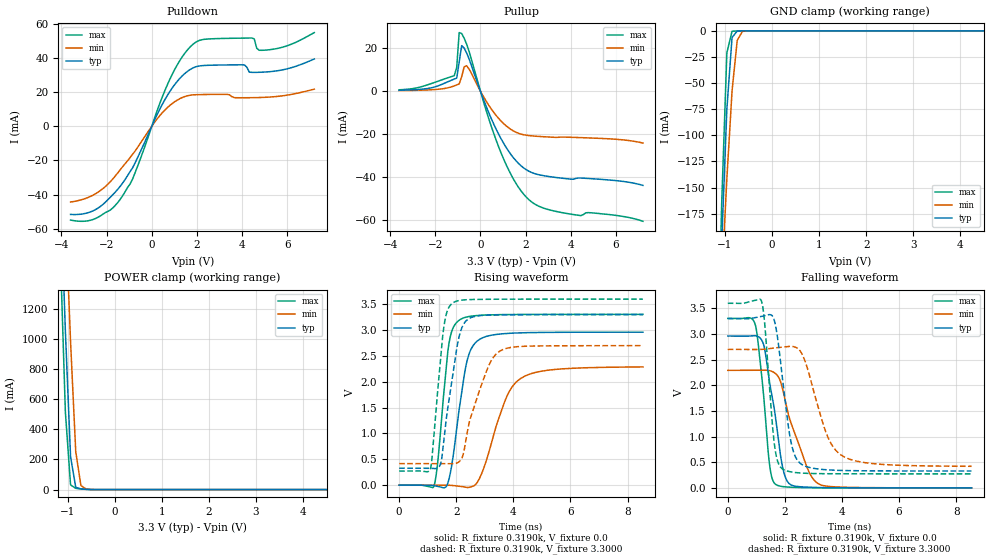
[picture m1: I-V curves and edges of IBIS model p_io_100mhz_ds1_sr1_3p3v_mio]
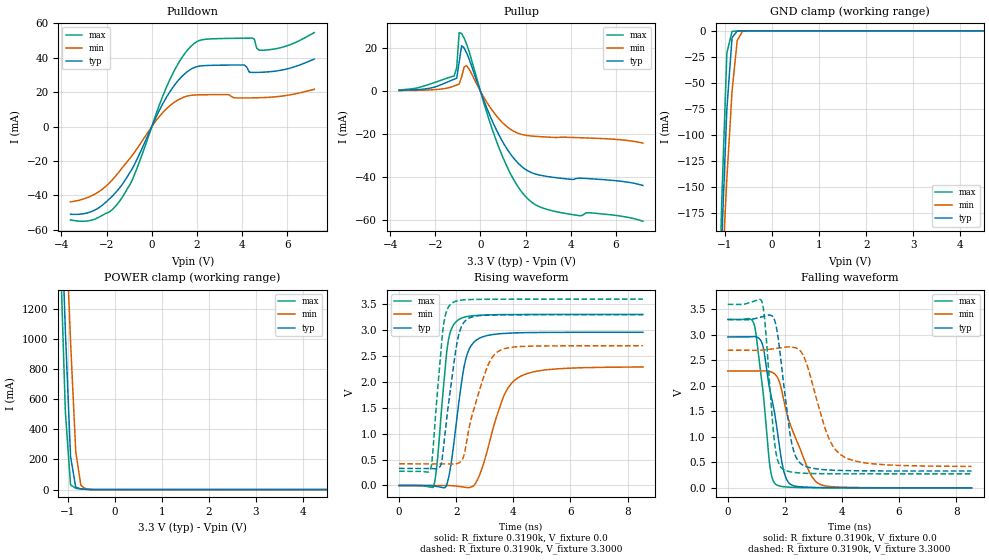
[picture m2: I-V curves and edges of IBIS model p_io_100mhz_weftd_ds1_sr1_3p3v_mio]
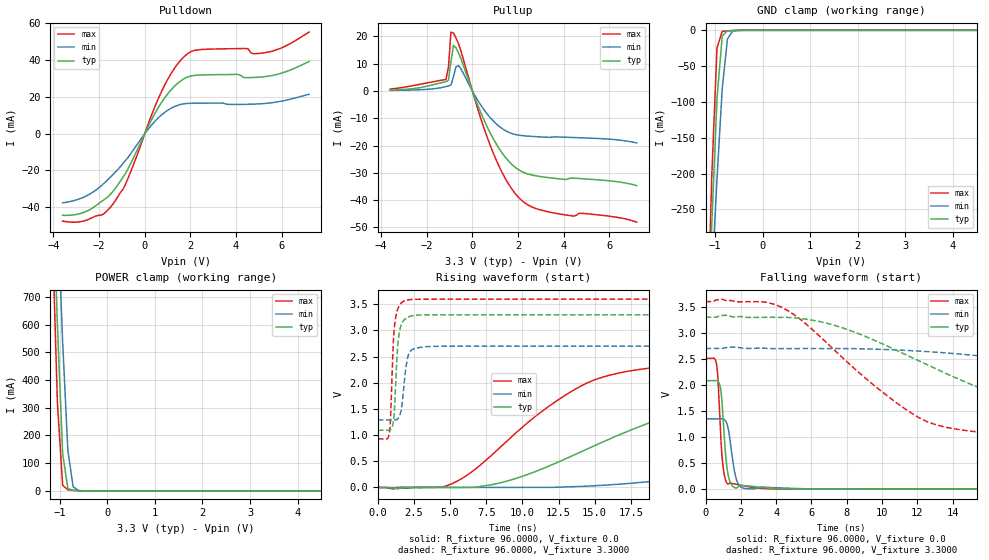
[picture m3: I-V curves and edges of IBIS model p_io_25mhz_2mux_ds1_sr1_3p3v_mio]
| IBIS file was generated by Viper version: 2025.10.06
[IBIS Ver]   6.0
[Comment Char]   |_char
[File Name]   c15x_c05x_32qfn.ibs
[File Rev]   1.0
[Date]   Wed Oct 22 17:23:39 2025
[Source]   NXP Viper 2025.10.06
[Notes]
[Disclaimer] IMPORTANT NOTICE
  This information is provided on an AS IS basis and without warranty.
  IN NO EVENT SHALL NXP BE LIABLE FOR INCIDENTAL OR CONSEQUENTIAL
  DAMAGES ARISING FROM USE OF THIS INFORMATION. THIS DISCLAIMER OF
  WARRANTY EXTENDS TO THE USER OF THE INFORMATION, AND TO THEIR CUSTOMERS
  OR USERS OF PRODUCTS  AND IS IN LIEU OF ALL WARRANTIES WHETHER EXPRESS,
  IMPLIED, OR STATUTORY, INCLUDING IMPLIED WARRANTIES OF MERCHANTABILITY
  OR FITNESS FOR PARTICULAR PURPOSE.
  NXP does not represent or warrant that the information furnished
  hereunder is free of infringement of any third party patents,
  copyrights, trade secrets, or other intellectual property rights.
  NXP does not represent or warrant that the information is free of
  defect, or that it meets any particular standard, requirements or need
  of the user of the infomation or their customers.
  NXP reserves the right to change the information in this file
  without notice.
   http://www.nxp.com
[Copyright]   (C) Copyright NXP 2004 - 2025, All Rights Reserved.
|   C15x_C05x_32QFN
[Component]   C15x_C05x_32QFN
[Manufacturer]   NXP
[Package]
| variable   typ   min   max
R_pkg   0.17548   0.155   0.21262
L_pkg   1.829e-09   1.531e-09   2.180e-09
C_pkg   1.363e-13   1.228e-13   1.594e-13
[Pin] signal_name   model_name   R_pin   L_pin   C_pin
1   P1_8   a_ip_io_3v_3p3v   0.19586   2.033e-09 1.444e-13
2   P1_9   a_ip_io_3v_3p3v   0.16891   1.839e-09 1.304e-13
3   P1_29   a_ip_io_3v_3p3v   0.15743   1.690e-09 1.249e-13
4   P1_30   a_ip_io_3v_3p3v   0.1554   1.610e-09 1.266e-13
5   P1_31   a_ip_io_3v_3p3v   0.1671   1.531e-09 1.394e-13
6   VDD_ANA   POWER   NA   NA   NA
7   VDD   POWER   NA   NA   NA
8   P2_2   a_ip_io_3v_3p3v   0.20204   2.076e-09 1.443e-13
9   P2_3   a_ip_io_3v_3p3v   0.18652   2.023e-09 1.375e-13
10   P2_7   a_ip_io_3v_3p3v   0.17002   1.817e-09 1.358e-13
11   P2_12   a_ip_io_3v_3p3v   0.16167   1.626e-09 1.309e-13
12   P2_13   a_ip_io_3v_3p3v   0.16236   1.566e-09 1.312e-13
13   P2_16   a_ip_io_3v_3p3v   0.16285   1.730e-09 1.317e-13
14   P2_17   a_ip_io_3v_3p3v   0.17748   1.921e-09 1.354e-13
15   P3_29   a_ip_io_3v_3p3v   0.17976   1.975e-09 1.316e-13
16   P3_28   a_ip_io_3v_3p3v   0.1962   2.019e-09 1.412e-13
17   P3_27   a_ip_io_3v_3p3v   0.21262   1.982e-09 1.525e-13
18   P3_11   a_ip_io_3v_3p3v   0.20043   2.180e-09 1.461e-13
19   P3_10   a_ip_io_3v_3p3v   0.17928   1.961e-09 1.401e-13
20   P3_9   a_ip_io_3v_3p3v   0.16389   1.788e-09 1.317e-13
21   P3_8   a_ip_io_3v_3p3v   0.1552   1.677e-09 1.278e-13
22   P3_1   a_ip_io_3v_3p3v   0.15887   1.668e-09 1.301e-13
23   P3_0   a_ip_io_3v_3p3v   0.1749   1.596e-09 1.442e-13
24   VDD   POWER   NA   NA   NA
25   P0_0   a_ip_io_3v_3p3v   0.19842   2.035e-09 1.483e-13
26   P0_1   a_ip_io_3v_3p3v   0.17716   1.923e-09 1.400e-13
27   P0_2   a_ip_io_3v_3p3v   0.1611   1.762e-09 1.312e-13
28   P0_3   a_ip_io_3v_3p3v   0.15523   1.732e-09 1.229e-13
29   P1_0   a_ip_io_3v_3p3v   0.155   1.701e-09 1.228e-13
30   P1_1   a_ip_io_3v_3p3v   0.16149   1.745e-09 1.302e-13
31   P1_2   a_ip_io_3v_3p3v   0.17972   1.876e-09 1.400e-13
32   P1_3   a_ip_io_3v_3p3v   0.21209   1.954e-09 1.594e-13
33   VSS   GND   NA   NA   NA
[Pin Mapping]   pulldown_ref   pullup_ref
1   VSS   VDD
2   VSS   VDD
3   VSS   VDD
4   VSS   VDD
5   VSS   VDD
6   NC   VDD_ANA
7   NC   VDD
8   VSS   VDD
9   VSS   VDD
10   VSS   VDD
11   VSS   VDD
12   VSS   VDD
13   VSS   VDD
14   VSS   VDD
15   VSS   VDD
16   VSS   VDD
17   VSS   VDD
18   VSS   VDD
19   VSS   VDD
20   VSS   VDD
21   VSS   VDD
22   VSS   VDD
23   VSS   VDD
24   NC   VDD
25   VSS   VDD
26   VSS   VDD
27   VSS   VDD
28   VSS   VDD
29   VSS   VDD
30   VSS   VDD
31   VSS   VDD
32   VSS   VDD
33   VSS   NC
|*   Model Selector   *
[Model Selector] a_ip_io_3v_3p3v
p_io_25mhz_ds0_sr0_3p3v_mio   dse=0 sre=0 25mhz
p_io_25mhz_ds0_sr1_3p3v_mio   dse=0 sre=1 25mhz
p_io_25mhz_ds1_sr0_3p3v_mio   dse=1 sre=0 25mhz
p_io_25mhz_ds1_sr1_3p3v_mio   dse=1 sre=1 25mhz
p_io_25mhz_r40_ds0_sr0_3p3v_mio   dse=0 sre=0 25mhz_r40
p_io_25mhz_r40_ds0_sr1_3p3v_mio   dse=0 sre=1 25mhz_r40
p_io_25mhz_r40_ds1_sr0_3p3v_mio   dse=1 sre=0 25mhz_r40
p_io_25mhz_r40_ds1_sr1_3p3v_mio   dse=1 sre=1 25mhz_r40
p_io_50mhz_ds0_sr0_3p3v_mio   dse=0 sre=0 50mhz
p_io_50mhz_ds0_sr1_3p3v_mio   dse=0 sre=1 50mhz
p_io_50mhz_ds1_sr0_3p3v_mio   dse=1 sre=0 50mhz
p_io_50mhz_ds1_sr1_3p3v_mio   dse=1 sre=1 50mhz
p_io_25mhz_cap_ds0_sr0_3p3v_mio   dse=0 sre=0 25mhz_cap
p_io_25mhz_cap_ds0_sr1_3p3v_mio   dse=0 sre=1 25mhz_cap
p_io_25mhz_cap_ds1_sr0_3p3v_mio   dse=1 sre=0 25mhz_cap
p_io_25mhz_cap_ds1_sr1_3p3v_mio   dse=1 sre=1 25mhz_cap
p_io_25mhz_2mux_ds0_sr0_3p3v_mio   dse=0 sre=0 25mhz_2mux
p_io_25mhz_2mux_ds0_sr1_3p3v_mio   dse=0 sre=1 25mhz_2mux
p_io_25mhz_2mux_ds1_sr0_3p3v_mio   dse=1 sre=0 25mhz_2mux
p_io_25mhz_2mux_ds1_sr1_3p3v_mio   dse=1 sre=1 25mhz_2mux
p_io_100mhz_ds0_sr0_3p3v_mio   dse=0 sre=0 100mhz
p_io_100mhz_ds0_sr1_3p3v_mio   dse=0 sre=1 100mhz
p_io_100mhz_ds1_sr0_3p3v_mio   dse=1 sre=0 100mhz
p_io_100mhz_ds1_sr1_3p3v_mio   dse=1 sre=1 100mhz
p_io_100mhz_weftd_ds0_sr0_3p3v_mio   dse=0 sre=0 100mhz
p_io_100mhz_weftd_ds0_sr1_3p3v_mio   dse=0 sre=1 100mhz
p_io_100mhz_weftd_ds1_sr0_3p3v_mio   dse=1 sre=0 100mhz
p_io_100mhz_weftd_ds1_sr1_3p3v_mio   dse=1 sre=1 100mhz
p_io_i2c_ds00_ds10_sr0_3p3v_mio   dse0=0 dse1=0 sre=0 i2c
p_io_i2c_ds00_ds10_sr1_3p3v_mio   dse0=0 dse1=0 sre=1 i2c
p_io_i2c_ds00_ds11_sr0_3p3v_mio   dse0=0 dse1=1 sre=0 i2c
p_io_i2c_ds00_ds11_sr1_3p3v_mio   dse0=0 dse1=1 sre=1 i2c
p_io_i2c_ds01_ds10_sr0_3p3v_mio   dse0=1 dse1=0 sre=0 i2c
p_io_i2c_ds01_ds10_sr1_3p3v_mio   dse0=1 dse1=0 sre=1 i2c
p_io_i2c_ds01_ds11_sr0_3p3v_mio   dse0=1 dse1=1 sre=0 i2c
p_io_i2c_ds01_ds11_sr1_3p3v_mio   dse0=1 dse1=1 sre=1 i2c
p_io_i2c_i2c1_3p3v_mio   ipp_i2c_lv=1 i2c
p_io_i2cfmp_ds00_ds10_sr0_3p3v_mio   dse0=0 dse1=0 sre=0 i2cfmp
p_io_i2cfmp_ds00_ds10_sr1_3p3v_mio   dse0=0 dse1=0 sre=1 i2cfmp
p_io_i2cfmp_ds00_ds11_sr0_3p3v_mio   dse0=0 dse1=1 sre=0 i2cfmp
p_io_i2cfmp_ds00_ds11_sr1_3p3v_mio   dse0=0 dse1=1 sre=1 i2cfmp
p_io_i2cfmp_ds01_ds10_sr0_3p3v_mio   dse0=1 dse1=0 sre=0 i2cfmp
p_io_i2cfmp_ds01_ds10_sr1_3p3v_mio   dse0=1 dse1=0 sre=1 i2cfmp
p_io_i2cfmp_ds01_ds11_sr0_3p3v_mio   dse0=1 dse1=1 sre=0 i2cfmp
p_io_i2cfmp_ds01_ds11_sr1_3p3v_mio   dse0=1 dse1=1 sre=1 i2cfmp
p_io_i2cfmp_i2c1_3p3v_mio   ipp_i2c_lv=1 i2cfmp
p_io_rst_3p3v_mio   rst
p_io_rst_rx1p8v_3p3v_mio   rst
p_io_aon_3p3v_mio   rst
| End [Component] C15x_C05x_32QFN
| Models and submodels in the file (49): p_io_100mhz_ds0_sr0_3p3v_mio (I/O), p_io_100mhz_ds0_sr1_3p3v_mio (I/O), p_io_100mhz_ds1_sr0_3p3v_mio (I/O), p_io_100mhz_ds1_sr1_3p3v_mio (I/O), p_io_100mhz_weftd_ds0_sr0_3p3v_mio (I/O), p_io_100mhz_weftd_ds0_sr1_3p3v_mio (I/O), p_io_100mhz_weftd_ds1_sr0_3p3v_mio (I/O), p_io_100mhz_weftd_ds1_sr1_3p3v_mio (I/O), p_io_25mhz_2mux_ds0_sr0_3p3v_mio (I/O), p_io_25mhz_2mux_ds0_sr1_3p3v_mio (I/O), p_io_25mhz_2mux_ds1_sr0_3p3v_mio (I/O), p_io_25mhz_2mux_ds1_sr1_3p3v_mio (I/O), p_io_25mhz_cap_ds0_sr0_3p3v_mio (I/O), p_io_25mhz_cap_ds0_sr1_3p3v_mio (I/O), p_io_25mhz_cap_ds1_sr0_3p3v_mio (I/O), p_io_25mhz_cap_ds1_sr1_3p3v_mio (I/O), p_io_25mhz_ds0_sr0_3p3v_mio (I/O), p_io_25mhz_ds0_sr1_3p3v_mio (I/O), p_io_25mhz_ds1_sr0_3p3v_mio (I/O), p_io_25mhz_ds1_sr1_3p3v_mio (I/O), p_io_25mhz_r40_ds0_sr0_3p3v_mio (I/O), p_io_25mhz_r40_ds0_sr1_3p3v_mio (I/O), p_io_25mhz_r40_ds1_sr0_3p3v_mio (I/O), p_io_25mhz_r40_ds1_sr1_3p3v_mio (I/O), p_io_50mhz_ds0_sr0_3p3v_mio (I/O), p_io_50mhz_ds0_sr1_3p3v_mio (I/O), p_io_50mhz_ds1_sr0_3p3v_mio (I/O), p_io_50mhz_ds1_sr1_3p3v_mio (I/O), p_io_aon_3p3v_mio (I/O), p_io_i2c_ds00_ds10_sr0_3p3v_mio (I/O), p_io_i2c_ds00_ds10_sr1_3p3v_mio (I/O), p_io_i2c_ds00_ds11_sr0_3p3v_mio (I/O), p_io_i2c_ds00_ds11_sr1_3p3v_mio (I/O), p_io_i2c_ds01_ds10_sr0_3p3v_mio (I/O), p_io_i2c_ds01_ds10_sr1_3p3v_mio (I/O), p_io_i2c_ds01_ds11_sr0_3p3v_mio (I/O), p_io_i2c_ds01_ds11_sr1_3p3v_mio (I/O), p_io_i2c_i2c1_3p3v_mio (I/O), p_io_i2cfmp_ds00_ds10_sr0_3p3v_mio (I/O), p_io_i2cfmp_ds00_ds10_sr1_3p3v_mio (I/O), p_io_i2cfmp_ds00_ds11_sr0_3p3v_mio (I/O), p_io_i2cfmp_ds00_ds11_sr1_3p3v_mio (I/O), p_io_i2cfmp_ds01_ds10_sr0_3p3v_mio (I/O), p_io_i2cfmp_ds01_ds10_sr1_3p3v_mio (I/O), p_io_i2cfmp_ds01_ds11_sr0_3p3v_mio (I/O), p_io_i2cfmp_ds01_ds11_sr1_3p3v_mio (I/O), p_io_i2cfmp_i2c1_3p3v_mio (I/O), p_io_rst_3p3v_mio (I/O), p_io_rst_rx1p8v_3p3v_mio (I/O)
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[Model] p_io_100mhz_ds1_sr1_3p3v_mio
|   Model p_io_100mhz_ds1_sr1_3p3v_mio
| This model was characterised for following simulation conditions:
| External (pad) voltage:
|   - Typ: 3.3V,   - Min: 2.7V,   - Max: 3.6V
| Library cells for typ/min/max conditions are connected as defined below:
|  pad - External Pad
|  ipp_do_lv - Core Input
|  ipp_obe_lv - Output Buffer Enable
|  IOGC - NC
|  REFH3V3 - REFH3V3
|  REFL3V3 - REFL3V3
|  ZI - NC
|  abut_ncal_vddio[1] - vddio
|  abut_ncal_vddio[2] - vddio
|  abut_ncal_vddio[3] - vssio
|  abut_ncal_vddio[4] - vddio
|  abut_ncal_vddio[5] - vddio
|  abut_ncal_vddio[6] - vssio
|  abut_pcal_vddio[1] - vssio
|  abut_pcal_vddio[2] - vssio
|  abut_pcal_vddio[3] - vddio
|  abut_pcal_vddio[4] - vssio
|  abut_pcal_vddio[5] - vssio
|  abut_pcal_vddio[6] - vddio
|  ipp_do_1p8v - ipp_do_1p8v
|  ipp_dse_lv - vdd_lv
|  ipp_eftd_lv - NC
|  ipp_ina_mux_vddio - NC
|  ipp_ina_mux_vddio[0] - NC
|  ipp_ina_mux_vddio[1] - NC
|  ipp_ina_r0_vddio - NC
|  ipp_ina_r0a_vddio - NC
|  ipp_ina_r0b_vddio - NC
|  ipp_ina_r0c_vddio - NC
|  ipp_ina_r0d_vddio - NC
|  ipp_ina_r0e_vddio - NC
|  ipp_ina_r0f_vddio - NC
|  ipp_ina_r300_vddio - NC
|  ipp_ina_r300a_vddio - NC
|  ipp_ina_r300b_vddio - NC
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Model_type I/O
Polarity   Non-Inverting
Enable   Active-High
Vinl =   0.9900V
Vinh =   2.3100V
Vmeas =  1.6500V
Cref =   30.0000pF
Rref =   1.0000M
Vref =   3.3000V
C_comp   1.3234pF   1.2639pF   1.4076pF
|C_comp_pullup   0.6740pF   0.7057pF   0.6520pF
|C_comp_pulldown   0.5815pF   0.6343pF   0.5433pF
[Model Spec]
| variable   typ   min   max
Vinh   2.3100V   1.8900V   2.5200V
Vinl   0.9900V   0.8100V   1.0800V
[Temperature Range]   25.0000   0.1250k   -40.0000
[Voltage Range]   3.3000V   2.7000V   3.6000V
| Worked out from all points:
|   slope of the pulldown table from 0 to 0.495 V, typ, clamps not added: 36.6 ohm
|   slope of the pullup table from 0 to 0.495 V, typ, clamps not added: 37.7 ohm
|   GND clamp passes 1 mA (typ) near -0.75 V on its own axis
|   POWER clamp passes 1 mA (typ) near -0.55 V on its own axis
|   rising waveform, R_fixture 0.3190k, V_fixture 0.0: 20-80 % time 463ps typ, 832ps min, 328ps max; typ from 0 V to 2.96 V
|   rising waveform, R_fixture 0.3190k, V_fixture 3.3000: 20-80 % time 462ps typ, 748ps min, 321ps max; typ from 0.328 V to 3.3 V
|   falling waveform, R_fixture 0.3190k, V_fixture 0.0: 20-80 % time 473ps typ, 774ps min, 322ps max; typ from 2.96 V to 0 V
|   falling waveform, R_fixture 0.3190k, V_fixture 3.3000: 20-80 % time 407ps typ, 769ps min, 280ps max; typ from 3.3 V to 0.329 V
[Pulldown]
|Voltage   I(typ)   I(min)   I(max)
-3.6V     -51.52mA   -44.27mA   -54.81mA
-2.5V     -48.75mA   -39.51mA   -53.96mA
-1.4V     -35.12mA   -25.45mA   -42.73mA
-850mV    -24.27mA   -16.41mA   -30.84mA
800mV     20.29mA    12.16mA    27.43mA
1.35V     29.44mA    16.78mA    40.57mA
1.9V      34.5mA     18.39mA    48.67mA
4.1V      35.87mA    16.66mA    51.51mA
4.43V     31.5mA     16.69mA    51.59mA
4.65V     31.5mA     16.75mA    45.53mA
5.09V     31.75mA    16.96mA    44.55mA
7.2V      39.3mA     21.67mA    54.74mA
[Pullup]
|Voltage   I(typ)   I(min)   I(max)
-3.6V     391.8uA    234.9uA    605.7uA
-1.16V    5.604mA    2.419mA    7.14mA
-1.05V    6.055mA    2.871mA    11mA
-940mV    13.56mA    3.339mA    27.24mA
-830mV    21.15mA    6.685mA    26.82mA
-720mV    20.05mA    11.26mA    24.61mA
-610mV    17.74mA    11.81mA    21.86mA
820mV     -20.29mA   -12.86mA   -26.23mA
1.48V     -31.23mA   -18.63mA   -41.23mA
2.03V     -36.57mA   -20.53mA   -49.31mA
3.46V     -40.33mA   -21.49mA   -56.22mA
7.2V      -43.87mA   -24.17mA   -60.58mA
[GND_clamp]
|Voltage   I(typ)   I(min)   I(max)
-3.6V     -4.134A    -3.035A    -5.609A
-1.18V    -349.4mA   -343.6mA   -365.7mA
-1.07V    -202.9mA   -239.3mA   -165.2mA
-960mV    -74.83mA   -141.5mA   -21.03mA
-850mV    -6.389mA   -57.64mA   -383.3uA
-740mV    -222.1uA   -9.174mA   -124.1uA
-630mV    -55.93uA   -558.9uA   -58.07uA
7.2V      0A         0A         0A
[POWER_clamp]
|Voltage   I(typ)   I(min)   I(max)
-3.6V     24.54A     22.33A     26.93A
-1.16V    2.046A     2.721A     1.599A
-1.05V    1.052A     1.847A     514.4mA
-940mV    218.6mA    981.8mA    31.16mA
-830mV    15.1mA     252.4mA    8.462mA
-720mV    4.281mA    26.81mA    4.453mA
-610mV    1.717mA    3.626mA    1.66mA
7.2V      0A         0A         0A
[Ramp]
| variable   typ   min   max
dV/dt_r  1.7762/0.4627n   1.3728/0.8323n   1.9832/0.3278n
dV/dt_f  1.7828/0.4074n   1.3676/0.7690n   1.9962/0.2798n
R_load = 0.3190k
[Rising Waveform]
R_fixture= 0.3190k
V_fixture= 0.0
V_fixture_min= 0.0
V_fixture_max= 0.0
|time   V(typ)   V(min)   V(max)
0s        2.902nV    250nV      9.459nV
1.223ns   -10.89mV   -6.469uV   -14.68mV
1.367ns   -23.26mV   432.8uV    521.7mV
1.741ns   105.6mV    -943.7uV   2.727V
2.104ns   1.469V     -19.16mV   3.193V
2.362ns   2.366V     -44.86mV   3.254V
2.644ns   2.739V     -3.7mV     3.278V
3.78ns    2.936V     1.726V     3.302V
4.288ns   2.948V     2.075V     3.304V
8.54ns    2.96V      2.288V     3.305V
[Rising Waveform]
R_fixture= 0.3190k
V_fixture= 3.3000
V_fixture_min= 2.7000
V_fixture_max= 3.6000
|time   V(typ)   V(min)   V(max)
0s        328.4mV    417.4mV    273mV
1.095ns   327.1mV    417.3mV    314.6mV
1.431ns   382.4mV    418mV      2.336V
1.553ns   812.4mV    418.4mV    3.011V
1.88ns    2.147V     415.2mV    3.527V
2.089ns   2.846V     449mV      3.572V
2.297ns   3.149V     734.8mV    3.587V
2.949ns   3.286V     2.042V     3.597V
3.527ns   3.295V     2.594V     3.599V
8.54ns    3.3V       2.7V       3.6V
[Falling Waveform]
R_fixture= 0.3190k
V_fixture= 0.0
V_fixture_min= 0.0
V_fixture_max= 0.0
|time   V(typ)   V(min)   V(max)
0s        2.961V     2.292V     3.305V
969.3ps   2.966V     2.29V      3.171V
1.26ns    2.783V     2.295V     1.777V
1.471ns   2.038V     2.285V     420.1mV
1.688ns   1.313V     2.221V     63.57mV
1.9ns     459.6mV    1.975V     27.02mV
2.078ns   134.8mV    1.527V     16.67mV
2.798ns   12.69mV    370.4mV    3.524mV
3.163ns   6.584mV    83.26mV    1.82mV
8.54ns    86.29uV    287.2uV    52.59uV
[Falling Waveform]
R_fixture= 0.3190k
V_fixture= 3.3000
V_fixture_min= 2.7000
V_fixture_max= 3.6000
|time   V(typ)   V(min)   V(max)
0s        3.3V       2.7V       3.6V
1.18ns    3.345V     2.7V       3.643V
1.299ns   3.357V     2.705V     3.175V
1.639ns   3.248V     2.728V     824.4mV
1.919ns   2.115V     2.746V     368.1mV
2.245ns   816.2mV    2.759V     308.4mV
2.666ns   434.4mV    2.531V     285.8mV
3.46ns    352.5mV    1.052V     275.7mV
4ns       339.2mV    629.7mV    274.2mV
8.54ns    328.6mV    420.6mV    273.1mV
[Model] p_io_100mhz_weftd_ds1_sr1_3p3v_mio
|   Model p_io_100mhz_weftd_ds1_sr1_3p3v_mio
| This model was characterised for following simulation conditions:
| External (pad) voltage:
|   - Typ: 3.3V,   - Min: 2.7V,   - Max: 3.6V
| Library cells for typ/min/max conditions are connected as defined below:
|  pad - External Pad
|  ipp_do_lv - Core Input
|  ipp_obe_lv - Output Buffer Enable
|  IOGC - NC
|  REFH3V3 - REFH3V3
|  REFL3V3 - REFL3V3
|  ZI - NC
|  abut_ncal_vddio[1] - vddio
|  abut_ncal_vddio[2] - vddio
|  abut_ncal_vddio[3] - vssio
|  abut_ncal_vddio[4] - vddio
|  abut_ncal_vddio[5] - vddio
|  abut_ncal_vddio[6] - vssio
|  abut_pcal_vddio[1] - vssio
|  abut_pcal_vddio[2] - vssio
|  abut_pcal_vddio[3] - vddio
|  abut_pcal_vddio[4] - vssio
|  abut_pcal_vddio[5] - vssio
|  abut_pcal_vddio[6] - vddio
|  ipp_do_1p8v - ipp_do_1p8v
|  ipp_dse_lv - vdd_lv
|  ipp_eftd_lv - NC
|  ipp_ina_mux_vddio - NC
|  ipp_ina_mux_vddio[0] - NC
|  ipp_ina_mux_vddio[1] - NC
|  ipp_ina_r0_vddio - NC
|  ipp_ina_r0a_vddio - NC
|  ipp_ina_r0b_vddio - NC
|  ipp_ina_r0c_vddio - NC
|  ipp_ina_r0d_vddio - NC
|  ipp_ina_r0e_vddio - NC
|  ipp_ina_r0f_vddio - NC
|  ipp_ina_r300_vddio - NC
|  ipp_ina_r300a_vddio - NC
|  ipp_ina_r300b_vddio - NC
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Model_type I/O
Polarity   Non-Inverting
Enable   Active-High
Vinl =   0.9900V
Vinh =   2.3100V
Vmeas =  1.6500V
Cref =   30.0000pF
Rref =   1.0000M
Vref =   3.3000V
C_comp   1.3824pF   1.3233pF   1.4661pF
|C_comp_pullup   0.6942pF   0.7256pF   0.6724pF
|C_comp_pulldown   0.6072pF   0.6599pF   0.5691pF
[Model Spec]
| variable   typ   min   max
Vinh   2.3100V   1.8900V   2.5200V
Vinl   0.9900V   0.8100V   1.0800V
[Temperature Range]   25.0000   0.1250k   -40.0000
[Voltage Range]   3.3000V   2.7000V   3.6000V
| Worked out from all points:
|   slope of the pulldown table from 0 to 0.495 V, typ, clamps not added: 36.8 ohm
|   slope of the pullup table from 0 to 0.495 V, typ, clamps not added: 37.8 ohm
|   GND clamp passes 1 mA (typ) near -0.75 V on its own axis
|   POWER clamp passes 1 mA (typ) near -0.55 V on its own axis
|   rising waveform, R_fixture 0.3190k, V_fixture 0.0: 20-80 % time 437ps typ, 779ps min, 310ps max; typ from 0 V to 2.96 V
|   rising waveform, R_fixture 0.3190k, V_fixture 3.3000: 20-80 % time 419ps typ, 681ps min, 295ps max; typ from 0.33 V to 3.3 V
|   falling waveform, R_fixture 0.3190k, V_fixture 0.0: 20-80 % time 516ps typ, 821ps min, 360ps max; typ from 2.96 V to 0 V
|   falling waveform, R_fixture 0.3190k, V_fixture 3.3000: 20-80 % time 404ps typ, 756ps min, 278ps max; typ from 3.3 V to 0.33 V
[Pulldown]
|Voltage   I(typ)   I(min)   I(max)
-3.6V     -50.99mA   -43.76mA   -54.26mA
-2.5V     -48.39mA   -39.11mA   -53.69mA
-1.4V     -35.22mA   -25.46mA   -42.92mA
-850mV    -24.19mA   -16.4mA    -30.69mA
800mV     20.23mA    12.14mA    27.32mA
1.35V     29.37mA    16.76mA    40.44mA
1.9V      34.45mA    18.38mA    48.57mA
4.1V      35.83mA    16.68mA    51.45mA
4.43V     31.54mA    16.72mA    51.52mA
4.65V     31.54mA    16.77mA    45.56mA
5.09V     31.78mA    16.98mA    44.58mA
7.2V      39.32mA    21.7mA     54.71mA
[Pullup]
|Voltage   I(typ)   I(min)   I(max)
-3.6V     392.3uA    235.2uA    607.2uA
-1.16V    5.571mA    2.41mA     7.094mA
-1.05V    6.017mA    2.857mA    10.99mA
-940mV    13.55mA    3.321mA    27.21mA
-830mV    21.12mA    6.673mA    26.77mA
-720mV    20.02mA    11.25mA    24.57mA
-610mV    17.72mA    11.8mA     21.82mA
820mV     -20.27mA   -12.85mA   -26.19mA
1.48V     -31.2mA    -18.62mA   -41.17mA
2.03V     -36.53mA   -20.52mA   -49.25mA
3.46V     -40.29mA   -21.47mA   -56.15mA
7.2V      -43.77mA   -24.12mA   -60.4mA
[GND_clamp]
|Voltage   I(typ)   I(min)   I(max)
-3.6V     -4.179A    -3.084A    -5.65A
-1.18V    -350.3mA   -344.8mA   -366.5mA
-1.07V    -203.5mA   -240.3mA   -165.6mA
-960mV    -75.17mA   -142.1mA   -21.27mA
-850mV    -6.53mA    -58.02mA   -538.4uA
-740mV    -289.9uA   -9.332mA   -209.1uA
-630mV    -85.04uA   -601.4uA   -92.54uA
-300mV    -199.1nA   -1.25uA    -48.79nA
7.2V      0A         0A         0A
[POWER_clamp]
|Voltage   I(typ)   I(min)   I(max)
-3.6V     24.55A     22.33A     26.93A
-1.16V    2.047A     2.721A     1.599A
-1.05V    1.052A     1.848A     514.6mA
-940mV    218.8mA    982.2mA    31.26mA
-830mV    15.16mA    252.6mA    8.517mA
-720mV    4.307mA    26.88mA    4.483mA
-610mV    1.728mA    3.641mA    1.672mA
7.2V      0A         0A         0A
[Ramp]
| variable   typ   min   max
dV/dt_r  1.7760/0.4370n   1.3734/0.7794n   1.9829/0.3103n
dV/dt_f  1.7821/0.4039n   1.3673/0.7561n   1.9953/0.2776n
R_load = 0.3190k
[Rising Waveform]
R_fixture= 0.3190k
V_fixture= 0.0
V_fixture_min= 0.0
V_fixture_max= 0.0
|time   V(typ)   V(min)   V(max)
0s        3.011nV    251.5nV    9.8nV
1.206ns   -7.522mV   -184.8uV   -19.52mV
1.335ns   -19.53mV   138.3uV    458.1mV
1.699ns   73.68mV    511.5uV    2.716V
2.066ns   1.506V     -15.7mV    3.197V
2.297ns   2.357V     -33.82mV   3.254V
2.579ns   2.744V     -16.26mV   3.279V
3.663ns   2.937V     1.724V     3.302V
4.159ns   2.949V     2.079V     3.304V
8.54ns    2.96V      2.289V     3.305V
[Rising Waveform]
R_fixture= 0.3190k
V_fixture= 3.3000
V_fixture_min= 2.7000
V_fixture_max= 3.6000
|time   V(typ)   V(min)   V(max)
0s        329.6mV    418.3mV    274.4mV
1.109ns   328.4mV    418.1mV    324.6mV
1.42ns    356.5mV    418.8mV    2.349V
1.532ns   621.3mV    419.3mV    3.006V
1.841ns   2.037V     415.3mV    3.519V
2.046ns   2.811V     426.2mV    3.569V
2.252ns   3.139V     548mV      3.585V
2.984ns   3.288V     2.134V     3.597V
3.493ns   3.295V     2.597V     3.599V
8.54ns    3.3V       2.7V       3.6V
[Falling Waveform]
R_fixture= 0.3190k
V_fixture= 0.0
V_fixture_min= 0.0
V_fixture_max= 0.0
|time   V(typ)   V(min)   V(max)
0s        2.96V      2.291V     3.305V
934.7ps   2.967V     2.29V      3.188V
1.227ns   2.791V     2.294V     1.925V
1.473ns   1.923V     2.283V     435.9mV
1.698ns   1.264V     2.2V       62.87mV
1.909ns   461.1mV    1.863V     26.49mV
2.107ns   120.5mV    1.382V     15.31mV
2.819ns   11.96mV    356.5mV    3.259mV
3.189ns   6.067mV    80.38mV    1.687mV
8.54ns    88.34uV    282uV      53.95uV
[Falling Waveform]
R_fixture= 0.3190k
V_fixture= 3.3000
V_fixture_min= 2.7000
V_fixture_max= 3.6000
|time   V(typ)   V(min)   V(max)
0s        3.3V       2.7V       3.6V
1.198ns   3.354V     2.701V     3.648V
1.316ns   3.371V     2.707V     3.169V
1.651ns   3.271V     2.732V     830.4mV
1.922ns   2.201V     2.753V     371.2mV
2.259ns   831.2mV    2.76V      308.2mV
2.651ns   441.4mV    2.59V      287.4mV
3.467ns   352.7mV    1.074V     277mV
4.001ns   339.9mV    632.4mV    275.6mV
8.54ns    329.9mV    421.2mV    274.5mV
[Model] p_io_25mhz_2mux_ds1_sr1_3p3v_mio
|   Model p_io_25mhz_2mux_ds1_sr1_3p3v_mio
| This model was characterised for following simulation conditions:
| External (pad) voltage:
|   - Typ: 3.3V,   - Min: 2.7V,   - Max: 3.6V
| Library cells for typ/min/max conditions are connected as defined below:
|  pad - External Pad
|  ipp_do_lv - Core Input
|  ipp_obe_lv - Output Buffer Enable
|  IOGC - NC
|  REFH3V3 - REFH3V3
|  REFL3V3 - REFL3V3
|  ZI - NC
|  abut_ncal_vddio[1] - vddio
|  abut_ncal_vddio[2] - vddio
|  abut_ncal_vddio[3] - vssio
|  abut_ncal_vddio[4] - vddio
|  abut_ncal_vddio[5] - vddio
|  abut_ncal_vddio[6] - vssio
|  abut_pcal_vddio[1] - vssio
|  abut_pcal_vddio[2] - vssio
|  abut_pcal_vddio[3] - vddio
|  abut_pcal_vddio[4] - vssio
|  abut_pcal_vddio[5] - vssio
|  abut_pcal_vddio[6] - vddio
|  ipp_do_1p8v - ipp_do_1p8v
|  ipp_dse_lv - vdd_lv
|  ipp_eftd_lv - NC
|  ipp_ina_mux_vddio - NC
|  ipp_ina_mux_vddio[0] - NC
|  ipp_ina_mux_vddio[1] - NC
|  ipp_ina_r0_vddio - NC
|  ipp_ina_r0a_vddio - NC
|  ipp_ina_r0b_vddio - NC
|  ipp_ina_r0c_vddio - NC
|  ipp_ina_r0d_vddio - NC
|  ipp_ina_r0e_vddio - NC
|  ipp_ina_r0f_vddio - NC
|  ipp_ina_r300_vddio - NC
|  ipp_ina_r300a_vddio - NC
|  ipp_ina_r300b_vddio - NC
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Model_type I/O
Polarity   Non-Inverting
Enable   Active-High
Vinl =   0.9900V
Vinh =   2.3100V
Vmeas =  1.6500V
Cref =   30.0000pF
Rref =   1.0000M
Vref =   3.3000V
C_comp   1.2811pF   1.2303pF   1.3501pF
|C_comp_pullup   0.5368pF   0.5680pF   0.5155pF
|C_comp_pulldown   0.6706pF   0.7073pF   0.6415pF
[Model Spec]
| variable   typ   min   max
Vinh   2.3100V   1.8900V   2.5200V
Vinl   0.9900V   0.8100V   1.0800V
[Temperature Range]   25.0000   0.1250k   -40.0000
[Voltage Range]   3.3000V   2.7000V   3.6000V
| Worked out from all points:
|   slope of the pulldown table from 0 to 0.495 V, typ, clamps not added: 40.8 ohm
|   slope of the pullup table from 0 to 0.495 V, typ, clamps not added: 47.8 ohm
|   GND clamp passes 1 mA (typ) near -0.74 V on its own axis
|   POWER clamp passes 1 mA (typ) near -0.62 V on its own axis
|   rising waveform, R_fixture 96.0000, V_fixture 0.0: 20-80 % time 12ns typ, 25.5ns min, 7.17ns max; typ from 0 V to 2.08 V
|   rising waveform, R_fixture 96.0000, V_fixture 3.3000: 20-80 % time 277ps typ, 348ps min, 248ps max; typ from 1.09 V to 3.3 V
|   falling waveform, R_fixture 96.0000, V_fixture 0.0: 20-80 % time 280ps typ, 355ps min, 248ps max; typ from 2.08 V to 0 V
|   falling waveform, R_fixture 96.0000, V_fixture 3.3000: 20-80 % time 9.25ns typ, 20.1ns min, 5.6ns max; typ from 3.3 V to 1.09 V
[Pulldown]
|Voltage   I(typ)   I(min)   I(max)
-3.6V     -44.37mA   -37.58mA   -47.51mA
-2.5V     -41.88mA   -33.45mA   -46.76mA
-1.84V    -36.35mA   -27.58mA   -43.92mA
-1.4V     -31.43mA   -22.29mA   -38.34mA
-850mV    -21.79mA   -14.63mA   -27.74mA
800mV     18.21mA    10.89mA    24.66mA
1.35V     26.41mA    15.03mA    36.45mA
1.9V      30.96mA    16.49mA    43.73mA
4.43V     30.52mA    16mA       46.39mA
4.76V     30.6mA     16.11mA    43.53mA
5.31V     31.15mA    16.53mA    44.19mA
7.2V      39.28mA    21.46mA    55.3mA
[Pullup]
|Voltage   I(typ)   I(min)   I(max)
-3.6V     375uA      207.1uA    721uA
-1.16V    3.419mA    1.608mA    4.218mA
-1.05V    3.929mA    1.825mA    8.684mA
-940mV    10.66mA    2.209mA    21.58mA
-830mV    16.7mA     5.227mA    21.23mA
-720mV    15.82mA    8.86mA     19.48mA
-610mV    14mA       9.299mA    17.3mA
820mV     -16.02mA   -10.13mA   -20.76mA
1.48V     -24.66mA   -14.68mA   -32.62mA
2.03V     -28.88mA   -16.19mA   -39.03mA
3.35V     -31.76mA   -16.97mA   -44.31mA
7.2V      -34.67mA   -19.04mA   -48.06mA
[GND_clamp]
|Voltage   I(typ)   I(min)   I(max)
-3.6V     -5.309A    -4.128A    -6.876A
-1.18V    -466mA     -495.4mA   -458.9mA
-1.07V    -271.1mA   -348.5mA   -204.6mA
-960mV    -95.65mA   -208mA     -24.74mA
-850mV    -8.096mA   -81.85mA   -1.471mA
-740mV    -719.7uA   -12.14mA   -717.6uA
-630mV    -272.5uA   -923.5uA   -300.8uA
-300mV    -385.6nA   -2.502uA   -74.88nA
7.2V      0A         0A         0A
[POWER_clamp]
|Voltage   I(typ)   I(min)   I(max)
-3.6V     14.48A     12.95A     16.35A
-1.16V    1.177A     1.535A     951.2mA
-1.05V    598.4mA    1.032A     318mA
-940mV    134.2mA    537.3mA    20.02mA
-830mV    8.708mA    145.4mA    4.242mA
-720mV    2.127mA    15.38mA    2.218mA
-610mV    847.4uA    1.853mA    834.1uA
7.2V      0A         0A         0A
[Ramp]
| variable   typ   min   max
dV/dt_r  1.2491/12.0373n   0.8026/25.5375n   1.5061/7.1717n
dV/dt_f  1.3249/9.2469n   0.8437/20.0855n   1.6024/5.6005n
R_load = 96.0000
[Rising Waveform]
R_fixture= 96.0000
V_fixture= 0.0
V_fixture_min= 0.0
V_fixture_max= 0.0
|time   V(typ)   V(min)   V(max)
0s        3.081nV    103.2nV    10.53nV
4.572ns   -81.02uV   -467uV     15.01mV
8.528ns   91.84mV    7.678uV    783.2mV
11.66ns   388.3mV    693.5uV    1.518V
14.79ns   773.2mV    29.16mV    2.034V
21.68ns   1.514V     196.4mV    2.356V
30.99ns   1.882V     534.2mV    2.456V
42.83ns   2.003V     937.6mV    2.493V
53.59ns   2.045V     1.127V     2.504V
127.4ns   2.082V     1.338V     2.51V
[Rising Waveform]
R_fixture= 96.0000
V_fixture= 3.3000
V_fixture_min= 2.7000
V_fixture_max= 3.6000
|time   V(typ)   V(min)   V(max)
0s        1.092V     1.289V     929.3mV
803.7ps   1.091V     1.289V     1.056V
872.4ps   1.1V       1.289V     1.314V
1.015ns   1.184V     1.289V     2.498V
1.097ns   1.316V     1.289V     2.918V
1.292ns   2.356V     1.295V     3.338V
1.568ns   3.069V     1.427V     3.511V
1.994ns   3.242V     2.393V     3.581V
2.277ns   3.276V     2.615V     3.592V
127.4ns   3.3V       2.7V       3.6V
[Falling Waveform]
R_fixture= 96.0000
V_fixture= 0.0
V_fixture_min= 0.0
V_fixture_max= 0.0
|time   V(typ)   V(min)   V(max)
0s        2.082V     1.348V     2.51V
628.2ps   2.085V     1.348V     2.384V
708.8ps   2.074V     1.348V     2.079V
818ps     1.982V     1.349V     1.278V
939ps     1.639V     1.351V     605.9mV
1.186ns   491mV      1.275V     128.8mV
1.432ns   107.4mV    825.9mV    118.9mV
1.862ns   47.89mV    93.5mV     85.59mV
3.337ns   26.85mV    36.7mV     11.08mV
127.4ns   207.6nV    4.315uV    21.7nV
[Falling Waveform]
R_fixture= 96.0000
V_fixture= 3.3000
V_fixture_min= 2.7000
V_fixture_max= 3.6000
|time   V(typ)   V(min)   V(max)
0s        3.3V       2.7V       3.6V
4.021ns   3.299V     2.697V     3.533V
7.321ns   3.144V     2.699V     2.663V
12.47ns   2.401V     2.643V     1.309V
17.53ns   1.677V     2.485V     1.041V
20.23ns   1.426V     2.369V     999.6mV
25.11ns   1.263V     2.136V     963.4mV
35.51ns   1.154V     1.674V     938.8mV
45.7ns    1.119V     1.476V     932.6mV
127.4ns   1.092V     1.294V     929.3mV
